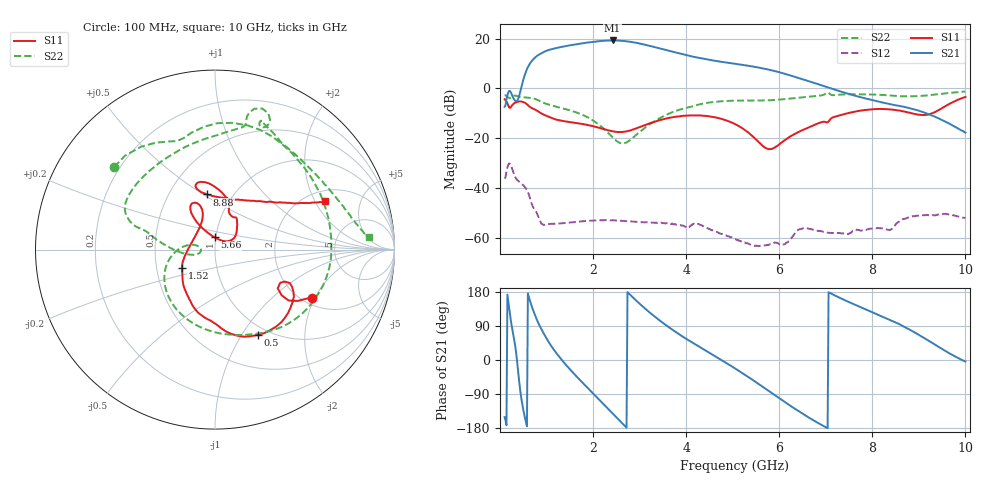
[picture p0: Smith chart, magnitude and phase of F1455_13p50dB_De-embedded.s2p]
! Integrated Device Technology
! Corporate Headquarters
! 6024 Silver Creek Valley Road
! San Jose, CA 95138  USA
! Phone:  1-408-284-8200
! Toll Free:  1-800-223-1366
! Webpage:  http://www.idt.com/
! Timing and RF Division
! 515 Groton Road, Suite 102
! Westford, MA 01886-6024
! Device:  F1455
! Description: 6-bit 0.5 dB Transmit Variable Gain Amplifier
! Frequency:  1400.0 -  2300.00 MHz
! Package:  6x6 mm Thin QFN Plastic Package: 28 pin
! State:  27
! Atten State:  13.5 dB
! Voltage:  +5.00 Volts
! Current:  217.632 mA
! Data:  The device was measured on a the F1455 evaluation board which has
!  individual transmission lines to the RF pins.  Data was collected
!  using a calibrated network analyzer.  The evaluation board was
!  de-embedded using a TRL calibration technique.
!  The reference plane is the edge of the package pin.
!  Pin  1 = CSb
!  Pin  2 = DATA
!  Pin  3 = CLK
!  Pin  4 = RSET
!  Pin  5 = GND
!  Pin  6 = RFIN  = Port 1
!  Pin  7 = GND
!  Pin  8 = NC
!  Pin  9 = NC
!  Pin 10 = NC
!  Pin 11 = NC
!  Pin 12 = NC
!  Pin 13 = NC
!  Pin 14 = /STBY
!  Pin 15 = GND
!  Pin 16 = RFOUT  = Port 2
!  Pin 17 = GND
!  Pin 18 = NC
!  Pin 19 = NC
!  Pin 20 = NC
!  Pin 21 = GND
!  Pin 22 = NC
!  Pin 23 = GND
!  Pin 24 = NC
!  Pin 25 = NC
!  Pin 26 = NC
!  Pin 27 = GND
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# GHz S dB R 50
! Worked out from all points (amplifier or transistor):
!   496 points, 100 MHz to 10 GHz, reference 50 ohm
!   highest |S21| = 19.3 dB at 2.42 GHz (marker M1)
!   |S21| within 3 dB of that: 1.221 GHz to 3.395 GHz (2.173 GHz wide, 94.2 % of centre)
!   unconditionally stable (mu >= 1): start of sweep to end of sweep
!   at 1.74 GHz: K = 25.63, MAG = 18.6 dB, |S12| = -53.4 dB
!   at 5.06 GHz: K = 112.36, MAG = 11.7 dB, |S12| = -60.6 dB
!   at 10 GHz: K = 217.80, MAG = -9.2 dB, |S12| = -52.1 dB
!   S11 on the Smith chart (normalised r, x): 100 MHz: 2.24, -1.90; 500 MHz: 0.89, -1.18; 1.52 GHz: 0.68, -0.14; 5.66 GHz: 0.99, +0.14; 8.88 GHz: 0.76, +0.52; 10 GHz: 2.48, +2.44
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0.1  -4.37 -26.4  -7.40 -150.7  -36.24 45.9  -2.78 140.7
0.24  -7.38 -24.6  -1.81 98.9  -31.16 -63.1  -3.55 101.3
0.38  -5.37 -40.7  -4.73 -17.9  -36.93 -114.1  -3.15 57.2
0.5  -5.49 -63.5  3.38 -130.7  -38.94 -152.2  -3.56 27.7
0.68  -7.86 -91.7  10.89 142.7  -46.21 144.4  -3.87 -13.8
0.94  -10.54 -121.1  14.61 70.1  -54.82 125.0  -5.82 -67.6
1.22  -12.58 -140.6  16.25 16.9  -54.33 99.6  -7.39 -107.2
1.52  -13.58 -151.5  17.36 -26.8  -53.87 71.4  -8.91 -138.6
1.76  -14.23 -158.4  18.08 -58.1  -53.36 53.4  -10.52 -158.4
2.1  -15.69 -171.7  18.91 -100.5  -53.01 32.3  -14.19 178.0
2.42  -17.23 166.2  19.26 -140.9  -52.99 14.1  -19.66 167.5
2.62  -17.54 146.6  19.12 -166.1  -53.21 4.7  -22.15 -179.6
2.8  -16.87 130.2  18.72 171.8  -53.42 -2.8  -20.68 -166.8
3.1  -14.85 113.2  17.61 137.6  -53.84 -13.6  -16.09 -171.1
3.4  -12.93 108.1  16.23 107.4  -53.99 -24.3  -12.35 178.6
4.1  -10.86 114.4  12.92 48.5  -55.04 -42.1  -7.39 164.3
5.06  -14.42 123.7  9.86 -22.8  -60.58 -84.2  -4.93 149.0
5.66  -23.32 91.9  8.00 -71.9  -63.14 -75.2  -4.84 124.7
6.7  -15.17 45.4  2.53 -156.6  -56.61 -131.2  -3.23 78.8
8.36  -8.40 106.1  -6.27 106.7  -56.89 159.6  -2.82 62.7
8.88  -10.15 98.1  -8.31 74.8  -51.37 144.7  -3.18 42.2
10  -3.46 23.7  -17.79 -3.9  -52.11 67.3  -1.27 4.7
